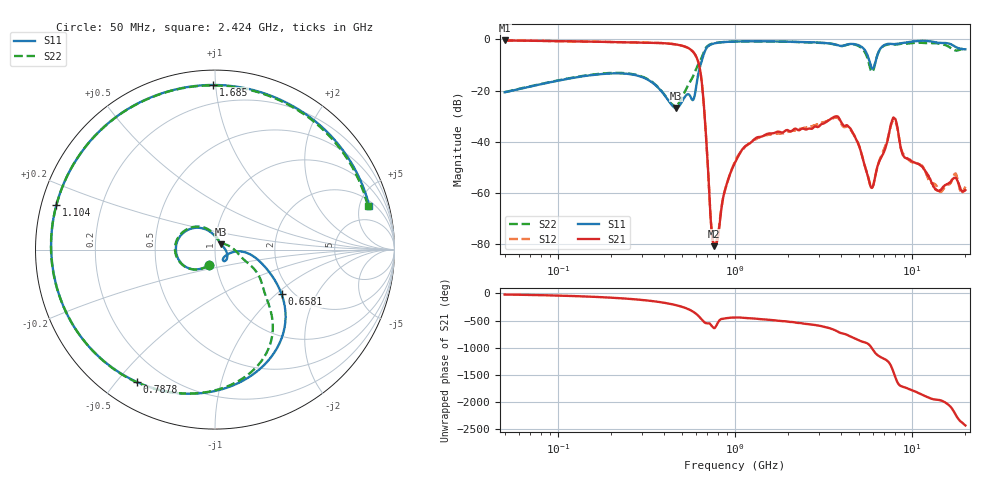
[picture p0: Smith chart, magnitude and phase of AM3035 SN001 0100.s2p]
# Hz S DB R 50
!freq MagS11 AngS11 MagS21 AngS21 MagS12 AngS12 MagS22 AngS22
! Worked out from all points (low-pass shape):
!   1601 points, 50 MHz to 20.05 GHz, reference 50 ohm
!   highest |S21| = -0.38 dB at 50 MHz (marker M1); lowest = -80.8 dB at 764.5 MHz (marker M2)
!   |S21| within 3 dB of the highest: start of sweep to 546.4 MHz
!   lowest |S11| = -26.8 dB at 464.5 MHz (marker M3), VSWR 1.10, Z = 53.4 + j3.27 ohm
!   |S11| at or under -10 dB: start of sweep to 639 MHz; 5.837 GHz to 6.151 GHz (314.2 MHz wide, 5.24 % of centre)
!   |S22| runs from -25.9 to -0.7 dB; largest |S21 - S12| = 0.0042
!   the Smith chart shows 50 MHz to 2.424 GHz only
!   S11 on the Smith chart (normalised r, x): 50 MHz: 0.92, -0.16; 658.1 MHz: 1.75, -1.08; 787.8 MHz: 0.10, -0.57; 1.104 GHz: 0.04, +0.14; 1.685 GHz: 0.09, +0.98; 2.424 GHz: 2.53, +6.13
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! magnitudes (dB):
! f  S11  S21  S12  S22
! 50 MHz  -20.6  -0.4  -0.4  -20.6
! 135.9 MHz  -14.4  -0.8  -0.8  -14.3
! 369.6 MHz  -18.9  -1.3  -1.4  -18.7
! 464.5 MHz  -26.8  -1.9  -1.9  -25.8
! 599.3 MHz  -20.0  -6.2  -6.2  -12.1
! 658.1 MHz  -7.0  -20.5  -20.5  -6.0
! 733.7 MHz  -1.9  -72.5  -72.0  -1.8
! 764.5 MHz  -1.5  -80.8  -80.3  -1.4
! 787.8 MHz  -1.3  -79.6  -78.3  -1.3
! 874.9 MHz  -1.0  -59.3  -59.4  -1.0
! 1.005 GHz  -0.8  -47.9  -47.4  -0.8
! 1.104 GHz  -0.7  -42.9  -43.1  -0.7
! 1.685 GHz  -0.8  -36.4  -36.7  -0.8
! 2.424 GHz  -1.0  -34.8  -34.7  -1.1
! 2.722 GHz  -1.1  -34.9  -34.0  -1.2
! 4.397 GHz  -1.8  -34.2  -34.5  -1.9
! 5.912 GHz  -11.0  -58.0  -58.0  -12.5
! 7.402 GHz  -1.7  -37.1  -37.2  -1.9
! 8.008 GHz  -1.8  -30.9  -31.9  -2.0
! 9.028 GHz  -1.3  -45.8  -45.2  -1.6
! 14.37 GHz  -1.3  -59.0  -59.4  -1.6
! 20.05 GHz  -3.8  -58.9  -57.5  -3.6
